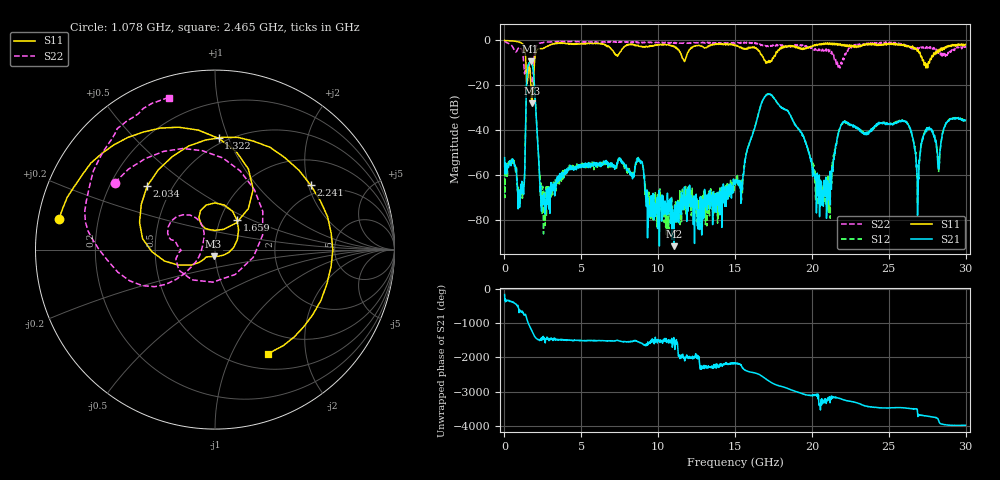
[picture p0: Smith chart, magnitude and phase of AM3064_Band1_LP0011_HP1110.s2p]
# Hz S DB R 50.0
!freq dBS11 angS11 dBS21 angS21 dBS12 angS12 dBS22 angS22
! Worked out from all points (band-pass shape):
!   1600 points, 10 MHz to 29.98 GHz, reference 50 ohm
!   highest |S21| = -9.41 dB at 1.697 GHz (marker M1); lowest = -91.9 dB at 11.03 GHz (marker M2)
!   |S21| within 3 dB of the highest: 1.508 GHz to 1.852 GHz (343.7 MHz wide, 20.5 % of centre)
!   lowest |S11| = -28.1 dB at 1.791 GHz (marker M3), VSWR 1.08, Z = 49 - j3.77 ohm
!   |S11| at or under -10 dB: 1.393 GHz to 1.949 GHz (556.5 MHz wide, 33.3 % of centre); 27.28172 GHz to 27.35194 GHz (70.22 MHz wide, 0.257 % of centre); 27.36 GHz to 27.57 GHz (208.4 MHz wide, 0.759 % of centre)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
!   |S22| runs from -22.8 to -0.3 dB; largest |S21 - S12| = 0.0058
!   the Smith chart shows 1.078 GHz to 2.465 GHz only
!   S11 on the Smith chart (normalised r, x): 1.078 GHz: 0.06, +0.10; 1.322 GHz: 0.46, +0.92; 1.659 GHz: 1.20, +0.41; 2.034 GHz: 0.36, +0.35; 2.241 GHz: 1.70, +2.07; 2.465 GHz: 0.69, -1.40
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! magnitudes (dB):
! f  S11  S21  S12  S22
! 10 MHz  0.0  -52.3  -54.2  -0.3
! 1.078 GHz  -1.0  -67.0  -64.3  -3.5
! 1.322 GHz  -4.1  -58.1  -56.6  -14.8
! 1.659 GHz  -13.8  -9.6  -9.5  -12.5
! 1.697 GHz  -17.3  -9.4  -9.4  -15.1
! 1.791 GHz  -28.1  -10.3  -10.3  -22.1
! 2.034 GHz  -5.7  -30.1  -30.0  -3.3
! 2.241 GHz  -3.8  -54.8  -54.8  -1.5
! 2.465 GHz  -3.7  -69.9  -71.0  -1.1
! 5.015 GHz  -1.4  -55.6  -55.8  -0.7
! 8.782 GHz  -2.7  -54.1  -54.0  -0.8
! 10 GHz  -2.0  -76.7  -70.7  -0.9
! 11.03 GHz  -2.8  -91.9  -76.7  -1.2
! 15 GHz  -2.2  -64.4  -61.6  -1.2
! 17.16 GHz  -9.6  -23.9  -23.9  -2.8
! 19.99 GHz  -2.8  -55.0  -56.5  -3.3
! 21.04 GHz  -1.4  -68.0  -60.7  -3.8
! 21.98 GHz  -1.8  -37.0  -37.0  -9.5
! 25 GHz  -1.3  -37.5  -37.2  -1.1
! 26.91 GHz  -4.2  -66.5  -62.6  -4.0
! 27.49 GHz  -10.9  -39.5  -39.4  -3.2
! 29.98 GHz  -1.7  -35.6  -36.0  -3.4
